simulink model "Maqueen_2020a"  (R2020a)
settings: Solver=VariableStepAuto  StartTime=0.0  StopTime=2  RelTol=1e-3
model workspace: external: MAT-File (data not in the file)
undefined symbols (not defined in the file or in its folder): deg, kg, m, mm, N, rad, s, smiData, X, Y, Z
libraries: sm_lib x459, fl_lib x12, nesl_utility x10
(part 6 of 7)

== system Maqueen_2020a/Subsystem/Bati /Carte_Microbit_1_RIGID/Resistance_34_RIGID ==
  ReferenceFrame : sm_lib/Frames and Transforms/Reference Frame
  Solid : sm_lib/Body Elements/File Solid  ExtGeomFileName=Resistance_Defaut_sldprt.STL  UnitType=Custom  ExtGeomFileUnits=mm  StepReaderType=HEX  ExportConvexHullGeometry=off  InertiaType=Custom  Mass=smiData.Solid(7).mass  MassUnits=kg  CenterOfMass=smiData.Solid(7).CoM  CenterOfMassUnits=mm  MomentsOfInertia=smiData.Solid(7).MoI  MomentsOfInertiaUnits=kg*mm^2  ProductsOfInertia=smiData.Solid(7).PoI  ProductsOfInertiaUnits=kg*mm^2  BasedOnType=Density  Density=1000  DensityUnits=kg/m^3  DoExposeReferenceFrame=on  SerializedFrames=<Frames/>  GraphicType=FromGeometry  MarkerShape=Sphere  MarkerSize=10  GraphicVisPropType=SimpleVisualProperties  GraphicDiffuseColor=smiData.Solid(7).color  GraphicSpecularColor=[0.5 0.5 0.5 1.0]  GraphicAmbientColor=[0.15 0.15 0.15 1.0]  GraphicEmissiveColor=[0.0 0.0 0.0 1.0]  GraphicShininess=75  GraphicOpacity=smiData.Solid(7).opacity
  F : PMIOPort  Side=Left
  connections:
  ReferenceFrame/RConn1 -- Solid/RConn1 -- F/RConn1

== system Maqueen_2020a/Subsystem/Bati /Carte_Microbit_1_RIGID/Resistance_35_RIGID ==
  ReferenceFrame : sm_lib/Frames and Transforms/Reference Frame
  Solid : sm_lib/Body Elements/File Solid  ExtGeomFileName=Resistance_Defaut_sldprt.STL  UnitType=Custom  ExtGeomFileUnits=mm  StepReaderType=HEX  ExportConvexHullGeometry=off  InertiaType=Custom  Mass=smiData.Solid(7).mass  MassUnits=kg  CenterOfMass=smiData.Solid(7).CoM  CenterOfMassUnits=mm  MomentsOfInertia=smiData.Solid(7).MoI  MomentsOfInertiaUnits=kg*mm^2  ProductsOfInertia=smiData.Solid(7).PoI  ProductsOfInertiaUnits=kg*mm^2  BasedOnType=Density  Density=1000  DensityUnits=kg/m^3  DoExposeReferenceFrame=on  SerializedFrames=<Frames/>  GraphicType=FromGeometry  MarkerShape=Sphere  MarkerSize=10  GraphicVisPropType=SimpleVisualProperties  GraphicDiffuseColor=smiData.Solid(7).color  GraphicSpecularColor=[0.5 0.5 0.5 1.0]  GraphicAmbientColor=[0.15 0.15 0.15 1.0]  GraphicEmissiveColor=[0.0 0.0 0.0 1.0]  GraphicShininess=75  GraphicOpacity=smiData.Solid(7).opacity
  F : PMIOPort  Side=Left
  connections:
  ReferenceFrame/RConn1 -- Solid/RConn1 -- F/RConn1

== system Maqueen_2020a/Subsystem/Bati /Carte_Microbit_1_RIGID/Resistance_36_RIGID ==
  ReferenceFrame : sm_lib/Frames and Transforms/Reference Frame
  Solid : sm_lib/Body Elements/File Solid  ExtGeomFileName=Resistance_Defaut_sldprt.STL  UnitType=Custom  ExtGeomFileUnits=mm  StepReaderType=HEX  ExportConvexHullGeometry=off  InertiaType=Custom  Mass=smiData.Solid(7).mass  MassUnits=kg  CenterOfMass=smiData.Solid(7).CoM  CenterOfMassUnits=mm  MomentsOfInertia=smiData.Solid(7).MoI  MomentsOfInertiaUnits=kg*mm^2  ProductsOfInertia=smiData.Solid(7).PoI  ProductsOfInertiaUnits=kg*mm^2  BasedOnType=Density  Density=1000  DensityUnits=kg/m^3  DoExposeReferenceFrame=on  SerializedFrames=<Frames/>  GraphicType=FromGeometry  MarkerShape=Sphere  MarkerSize=10  GraphicVisPropType=SimpleVisualProperties  GraphicDiffuseColor=smiData.Solid(7).color  GraphicSpecularColor=[0.5 0.5 0.5 1.0]  GraphicAmbientColor=[0.15 0.15 0.15 1.0]  GraphicEmissiveColor=[0.0 0.0 0.0 1.0]  GraphicShininess=75  GraphicOpacity=smiData.Solid(7).opacity
  F : PMIOPort  Side=Left
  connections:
  ReferenceFrame/RConn1 -- Solid/RConn1 -- F/RConn1

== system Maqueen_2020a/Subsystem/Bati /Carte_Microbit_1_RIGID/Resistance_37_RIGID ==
  ReferenceFrame : sm_lib/Frames and Transforms/Reference Frame
  Solid : sm_lib/Body Elements/File Solid  ExtGeomFileName=Resistance_Defaut_sldprt.STL  UnitType=Custom  ExtGeomFileUnits=mm  StepReaderType=HEX  ExportConvexHullGeometry=off  InertiaType=Custom  Mass=smiData.Solid(7).mass  MassUnits=kg  CenterOfMass=smiData.Solid(7).CoM  CenterOfMassUnits=mm  MomentsOfInertia=smiData.Solid(7).MoI  MomentsOfInertiaUnits=kg*mm^2  ProductsOfInertia=smiData.Solid(7).PoI  ProductsOfInertiaUnits=kg*mm^2  BasedOnType=Density  Density=1000  DensityUnits=kg/m^3  DoExposeReferenceFrame=on  SerializedFrames=<Frames/>  GraphicType=FromGeometry  MarkerShape=Sphere  MarkerSize=10  GraphicVisPropType=SimpleVisualProperties  GraphicDiffuseColor=smiData.Solid(7).color  GraphicSpecularColor=[0.5 0.5 0.5 1.0]  GraphicAmbientColor=[0.15 0.15 0.15 1.0]  GraphicEmissiveColor=[0.0 0.0 0.0 1.0]  GraphicShininess=75  GraphicOpacity=smiData.Solid(7).opacity
  F : PMIOPort  Side=Left
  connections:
  ReferenceFrame/RConn1 -- Solid/RConn1 -- F/RConn1

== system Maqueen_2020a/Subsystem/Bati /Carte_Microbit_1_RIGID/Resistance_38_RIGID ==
  ReferenceFrame : sm_lib/Frames and Transforms/Reference Frame
  Solid : sm_lib/Body Elements/File Solid  ExtGeomFileName=Resistance_Defaut_sldprt.STL  UnitType=Custom  ExtGeomFileUnits=mm  StepReaderType=HEX  ExportConvexHullGeometry=off  InertiaType=Custom  Mass=smiData.Solid(7).mass  MassUnits=kg  CenterOfMass=smiData.Solid(7).CoM  CenterOfMassUnits=mm  MomentsOfInertia=smiData.Solid(7).MoI  MomentsOfInertiaUnits=kg*mm^2  ProductsOfInertia=smiData.Solid(7).PoI  ProductsOfInertiaUnits=kg*mm^2  BasedOnType=Density  Density=1000  DensityUnits=kg/m^3  DoExposeReferenceFrame=on  SerializedFrames=<Frames/>  GraphicType=FromGeometry  MarkerShape=Sphere  MarkerSize=10  GraphicVisPropType=SimpleVisualProperties  GraphicDiffuseColor=smiData.Solid(7).color  GraphicSpecularColor=[0.5 0.5 0.5 1.0]  GraphicAmbientColor=[0.15 0.15 0.15 1.0]  GraphicEmissiveColor=[0.0 0.0 0.0 1.0]  GraphicShininess=75  GraphicOpacity=smiData.Solid(7).opacity
  F : PMIOPort  Side=Left
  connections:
  ReferenceFrame/RConn1 -- Solid/RConn1 -- F/RConn1

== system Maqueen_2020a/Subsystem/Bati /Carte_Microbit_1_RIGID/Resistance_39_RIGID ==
  ReferenceFrame : sm_lib/Frames and Transforms/Reference Frame
  Solid : sm_lib/Body Elements/File Solid  ExtGeomFileName=Resistance_Defaut_sldprt.STL  UnitType=Custom  ExtGeomFileUnits=mm  StepReaderType=HEX  ExportConvexHullGeometry=off  InertiaType=Custom  Mass=smiData.Solid(7).mass  MassUnits=kg  CenterOfMass=smiData.Solid(7).CoM  CenterOfMassUnits=mm  MomentsOfInertia=smiData.Solid(7).MoI  MomentsOfInertiaUnits=kg*mm^2  ProductsOfInertia=smiData.Solid(7).PoI  ProductsOfInertiaUnits=kg*mm^2  BasedOnType=Density  Density=1000  DensityUnits=kg/m^3  DoExposeReferenceFrame=on  SerializedFrames=<Frames/>  GraphicType=FromGeometry  MarkerShape=Sphere  MarkerSize=10  GraphicVisPropType=SimpleVisualProperties  GraphicDiffuseColor=smiData.Solid(7).color  GraphicSpecularColor=[0.5 0.5 0.5 1.0]  GraphicAmbientColor=[0.15 0.15 0.15 1.0]  GraphicEmissiveColor=[0.0 0.0 0.0 1.0]  GraphicShininess=75  GraphicOpacity=smiData.Solid(7).opacity
  F : PMIOPort  Side=Left
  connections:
  ReferenceFrame/RConn1 -- Solid/RConn1 -- F/RConn1

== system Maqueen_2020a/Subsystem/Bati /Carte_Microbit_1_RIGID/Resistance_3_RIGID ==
  ReferenceFrame : sm_lib/Frames and Transforms/Reference Frame
  Solid : sm_lib/Body Elements/File Solid  ExtGeomFileName=Resistance_Defaut_sldprt.STL  UnitType=Custom  ExtGeomFileUnits=mm  StepReaderType=HEX  ExportConvexHullGeometry=off  InertiaType=Custom  Mass=smiData.Solid(7).mass  MassUnits=kg  CenterOfMass=smiData.Solid(7).CoM  CenterOfMassUnits=mm  MomentsOfInertia=smiData.Solid(7).MoI  MomentsOfInertiaUnits=kg*mm^2  ProductsOfInertia=smiData.Solid(7).PoI  ProductsOfInertiaUnits=kg*mm^2  BasedOnType=Density  Density=1000  DensityUnits=kg/m^3  DoExposeReferenceFrame=on  SerializedFrames=<Frames/>  GraphicType=FromGeometry  MarkerShape=Sphere  MarkerSize=10  GraphicVisPropType=SimpleVisualProperties  GraphicDiffuseColor=smiData.Solid(7).color  GraphicSpecularColor=[0.5 0.5 0.5 1.0]  GraphicAmbientColor=[0.15 0.15 0.15 1.0]  GraphicEmissiveColor=[0.0 0.0 0.0 1.0]  GraphicShininess=75  GraphicOpacity=smiData.Solid(7).opacity
  F : PMIOPort  Side=Left
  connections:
  ReferenceFrame/RConn1 -- Solid/RConn1 -- F/RConn1

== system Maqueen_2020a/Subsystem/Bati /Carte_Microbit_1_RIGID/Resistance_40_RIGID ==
  ReferenceFrame : sm_lib/Frames and Transforms/Reference Frame
  Solid : sm_lib/Body Elements/File Solid  ExtGeomFileName=Resistance_Defaut_sldprt.STL  UnitType=Custom  ExtGeomFileUnits=mm  StepReaderType=HEX  ExportConvexHullGeometry=off  InertiaType=Custom  Mass=smiData.Solid(7).mass  MassUnits=kg  CenterOfMass=smiData.Solid(7).CoM  CenterOfMassUnits=mm  MomentsOfInertia=smiData.Solid(7).MoI  MomentsOfInertiaUnits=kg*mm^2  ProductsOfInertia=smiData.Solid(7).PoI  ProductsOfInertiaUnits=kg*mm^2  BasedOnType=Density  Density=1000  DensityUnits=kg/m^3  DoExposeReferenceFrame=on  SerializedFrames=<Frames/>  GraphicType=FromGeometry  MarkerShape=Sphere  MarkerSize=10  GraphicVisPropType=SimpleVisualProperties  GraphicDiffuseColor=smiData.Solid(7).color  GraphicSpecularColor=[0.5 0.5 0.5 1.0]  GraphicAmbientColor=[0.15 0.15 0.15 1.0]  GraphicEmissiveColor=[0.0 0.0 0.0 1.0]  GraphicShininess=75  GraphicOpacity=smiData.Solid(7).opacity
  F : PMIOPort  Side=Left
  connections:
  ReferenceFrame/RConn1 -- Solid/RConn1 -- F/RConn1

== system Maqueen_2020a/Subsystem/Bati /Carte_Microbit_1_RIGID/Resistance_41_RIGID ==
  ReferenceFrame : sm_lib/Frames and Transforms/Reference Frame
  Solid : sm_lib/Body Elements/File Solid  ExtGeomFileName=Resistance_Defaut_sldprt.STL  UnitType=Custom  ExtGeomFileUnits=mm  StepReaderType=HEX  ExportConvexHullGeometry=off  InertiaType=Custom  Mass=smiData.Solid(7).mass  MassUnits=kg  CenterOfMass=smiData.Solid(7).CoM  CenterOfMassUnits=mm  MomentsOfInertia=smiData.Solid(7).MoI  MomentsOfInertiaUnits=kg*mm^2  ProductsOfInertia=smiData.Solid(7).PoI  ProductsOfInertiaUnits=kg*mm^2  BasedOnType=Density  Density=1000  DensityUnits=kg/m^3  DoExposeReferenceFrame=on  SerializedFrames=<Frames/>  GraphicType=FromGeometry  MarkerShape=Sphere  MarkerSize=10  GraphicVisPropType=SimpleVisualProperties  GraphicDiffuseColor=smiData.Solid(7).color  GraphicSpecularColor=[0.5 0.5 0.5 1.0]  GraphicAmbientColor=[0.15 0.15 0.15 1.0]  GraphicEmissiveColor=[0.0 0.0 0.0 1.0]  GraphicShininess=75  GraphicOpacity=smiData.Solid(7).opacity
  F : PMIOPort  Side=Left
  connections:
  ReferenceFrame/RConn1 -- Solid/RConn1 -- F/RConn1

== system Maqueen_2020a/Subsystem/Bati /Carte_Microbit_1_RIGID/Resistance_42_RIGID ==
  ReferenceFrame : sm_lib/Frames and Transforms/Reference Frame
  Solid : sm_lib/Body Elements/File Solid  ExtGeomFileName=Resistance_Defaut_sldprt.STL  UnitType=Custom  ExtGeomFileUnits=mm  StepReaderType=HEX  ExportConvexHullGeometry=off  InertiaType=Custom  Mass=smiData.Solid(7).mass  MassUnits=kg  CenterOfMass=smiData.Solid(7).CoM  CenterOfMassUnits=mm  MomentsOfInertia=smiData.Solid(7).MoI  MomentsOfInertiaUnits=kg*mm^2  ProductsOfInertia=smiData.Solid(7).PoI  ProductsOfInertiaUnits=kg*mm^2  BasedOnType=Density  Density=1000  DensityUnits=kg/m^3  DoExposeReferenceFrame=on  SerializedFrames=<Frames/>  GraphicType=FromGeometry  MarkerShape=Sphere  MarkerSize=10  GraphicVisPropType=SimpleVisualProperties  GraphicDiffuseColor=smiData.Solid(7).color  GraphicSpecularColor=[0.5 0.5 0.5 1.0]  GraphicAmbientColor=[0.15 0.15 0.15 1.0]  GraphicEmissiveColor=[0.0 0.0 0.0 1.0]  GraphicShininess=75  GraphicOpacity=smiData.Solid(7).opacity
  F : PMIOPort  Side=Left
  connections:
  ReferenceFrame/RConn1 -- Solid/RConn1 -- F/RConn1

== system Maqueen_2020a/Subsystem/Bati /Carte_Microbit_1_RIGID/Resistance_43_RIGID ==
  ReferenceFrame : sm_lib/Frames and Transforms/Reference Frame
  Solid : sm_lib/Body Elements/File Solid  ExtGeomFileName=Resistance_Defaut_sldprt.STL  UnitType=Custom  ExtGeomFileUnits=mm  StepReaderType=HEX  ExportConvexHullGeometry=off  InertiaType=Custom  Mass=smiData.Solid(7).mass  MassUnits=kg  CenterOfMass=smiData.Solid(7).CoM  CenterOfMassUnits=mm  MomentsOfInertia=smiData.Solid(7).MoI  MomentsOfInertiaUnits=kg*mm^2  ProductsOfInertia=smiData.Solid(7).PoI  ProductsOfInertiaUnits=kg*mm^2  BasedOnType=Density  Density=1000  DensityUnits=kg/m^3  DoExposeReferenceFrame=on  SerializedFrames=<Frames/>  GraphicType=FromGeometry  MarkerShape=Sphere  MarkerSize=10  GraphicVisPropType=SimpleVisualProperties  GraphicDiffuseColor=smiData.Solid(7).color  GraphicSpecularColor=[0.5 0.5 0.5 1.0]  GraphicAmbientColor=[0.15 0.15 0.15 1.0]  GraphicEmissiveColor=[0.0 0.0 0.0 1.0]  GraphicShininess=75  GraphicOpacity=smiData.Solid(7).opacity
  F : PMIOPort  Side=Left
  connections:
  ReferenceFrame/RConn1 -- Solid/RConn1 -- F/RConn1

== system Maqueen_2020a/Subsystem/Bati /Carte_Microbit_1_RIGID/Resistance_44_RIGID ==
  ReferenceFrame : sm_lib/Frames and Transforms/Reference Frame
  Solid : sm_lib/Body Elements/File Solid  ExtGeomFileName=Resistance_Defaut_sldprt.STL  UnitType=Custom  ExtGeomFileUnits=mm  StepReaderType=HEX  ExportConvexHullGeometry=off  InertiaType=Custom  Mass=smiData.Solid(7).mass  MassUnits=kg  CenterOfMass=smiData.Solid(7).CoM  CenterOfMassUnits=mm  MomentsOfInertia=smiData.Solid(7).MoI  MomentsOfInertiaUnits=kg*mm^2  ProductsOfInertia=smiData.Solid(7).PoI  ProductsOfInertiaUnits=kg*mm^2  BasedOnType=Density  Density=1000  DensityUnits=kg/m^3  DoExposeReferenceFrame=on  SerializedFrames=<Frames/>  GraphicType=FromGeometry  MarkerShape=Sphere  MarkerSize=10  GraphicVisPropType=SimpleVisualProperties  GraphicDiffuseColor=smiData.Solid(7).color  GraphicSpecularColor=[0.5 0.5 0.5 1.0]  GraphicAmbientColor=[0.15 0.15 0.15 1.0]  GraphicEmissiveColor=[0.0 0.0 0.0 1.0]  GraphicShininess=75  GraphicOpacity=smiData.Solid(7).opacity
  F : PMIOPort  Side=Left
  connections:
  ReferenceFrame/RConn1 -- Solid/RConn1 -- F/RConn1

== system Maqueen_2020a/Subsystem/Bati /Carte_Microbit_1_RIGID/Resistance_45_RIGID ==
  ReferenceFrame : sm_lib/Frames and Transforms/Reference Frame
  Solid : sm_lib/Body Elements/File Solid  ExtGeomFileName=Resistance_Defaut_sldprt.STL  UnitType=Custom  ExtGeomFileUnits=mm  StepReaderType=HEX  ExportConvexHullGeometry=off  InertiaType=Custom  Mass=smiData.Solid(7).mass  MassUnits=kg  CenterOfMass=smiData.Solid(7).CoM  CenterOfMassUnits=mm  MomentsOfInertia=smiData.Solid(7).MoI  MomentsOfInertiaUnits=kg*mm^2  ProductsOfInertia=smiData.Solid(7).PoI  ProductsOfInertiaUnits=kg*mm^2  BasedOnType=Density  Density=1000  DensityUnits=kg/m^3  DoExposeReferenceFrame=on  SerializedFrames=<Frames/>  GraphicType=FromGeometry  MarkerShape=Sphere  MarkerSize=10  GraphicVisPropType=SimpleVisualProperties  GraphicDiffuseColor=smiData.Solid(7).color  GraphicSpecularColor=[0.5 0.5 0.5 1.0]  GraphicAmbientColor=[0.15 0.15 0.15 1.0]  GraphicEmissiveColor=[0.0 0.0 0.0 1.0]  GraphicShininess=75  GraphicOpacity=smiData.Solid(7).opacity
  F : PMIOPort  Side=Left
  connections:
  ReferenceFrame/RConn1 -- Solid/RConn1 -- F/RConn1

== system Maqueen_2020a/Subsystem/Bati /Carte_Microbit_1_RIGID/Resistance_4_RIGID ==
  ReferenceFrame : sm_lib/Frames and Transforms/Reference Frame
  Solid : sm_lib/Body Elements/File Solid  ExtGeomFileName=Resistance_Defaut_sldprt.STL  UnitType=Custom  ExtGeomFileUnits=mm  StepReaderType=HEX  ExportConvexHullGeometry=off  InertiaType=Custom  Mass=smiData.Solid(7).mass  MassUnits=kg  CenterOfMass=smiData.Solid(7).CoM  CenterOfMassUnits=mm  MomentsOfInertia=smiData.Solid(7).MoI  MomentsOfInertiaUnits=kg*mm^2  ProductsOfInertia=smiData.Solid(7).PoI  ProductsOfInertiaUnits=kg*mm^2  BasedOnType=Density  Density=1000  DensityUnits=kg/m^3  DoExposeReferenceFrame=on  SerializedFrames=<Frames/>  GraphicType=FromGeometry  MarkerShape=Sphere  MarkerSize=10  GraphicVisPropType=SimpleVisualProperties  GraphicDiffuseColor=smiData.Solid(7).color  GraphicSpecularColor=[0.5 0.5 0.5 1.0]  GraphicAmbientColor=[0.15 0.15 0.15 1.0]  GraphicEmissiveColor=[0.0 0.0 0.0 1.0]  GraphicShininess=75  GraphicOpacity=smiData.Solid(7).opacity
  F : PMIOPort  Side=Left
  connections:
  ReferenceFrame/RConn1 -- Solid/RConn1 -- F/RConn1

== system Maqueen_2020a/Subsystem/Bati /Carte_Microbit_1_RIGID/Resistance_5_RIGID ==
  ReferenceFrame : sm_lib/Frames and Transforms/Reference Frame
  Solid : sm_lib/Body Elements/File Solid  ExtGeomFileName=Resistance_Defaut_sldprt.STL  UnitType=Custom  ExtGeomFileUnits=mm  StepReaderType=HEX  ExportConvexHullGeometry=off  InertiaType=Custom  Mass=smiData.Solid(7).mass  MassUnits=kg  CenterOfMass=smiData.Solid(7).CoM  CenterOfMassUnits=mm  MomentsOfInertia=smiData.Solid(7).MoI  MomentsOfInertiaUnits=kg*mm^2  ProductsOfInertia=smiData.Solid(7).PoI  ProductsOfInertiaUnits=kg*mm^2  BasedOnType=Density  Density=1000  DensityUnits=kg/m^3  DoExposeReferenceFrame=on  SerializedFrames=<Frames/>  GraphicType=FromGeometry  MarkerShape=Sphere  MarkerSize=10  GraphicVisPropType=SimpleVisualProperties  GraphicDiffuseColor=smiData.Solid(7).color  GraphicSpecularColor=[0.5 0.5 0.5 1.0]  GraphicAmbientColor=[0.15 0.15 0.15 1.0]  GraphicEmissiveColor=[0.0 0.0 0.0 1.0]  GraphicShininess=75  GraphicOpacity=smiData.Solid(7).opacity
  F : PMIOPort  Side=Left
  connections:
  ReferenceFrame/RConn1 -- Solid/RConn1 -- F/RConn1

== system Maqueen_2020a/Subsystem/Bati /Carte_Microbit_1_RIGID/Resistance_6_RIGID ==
  ReferenceFrame : sm_lib/Frames and Transforms/Reference Frame
  Solid : sm_lib/Body Elements/File Solid  ExtGeomFileName=Resistance_Defaut_sldprt.STL  UnitType=Custom  ExtGeomFileUnits=mm  StepReaderType=HEX  ExportConvexHullGeometry=off  InertiaType=Custom  Mass=smiData.Solid(7).mass  MassUnits=kg  CenterOfMass=smiData.Solid(7).CoM  CenterOfMassUnits=mm  MomentsOfInertia=smiData.Solid(7).MoI  MomentsOfInertiaUnits=kg*mm^2  ProductsOfInertia=smiData.Solid(7).PoI  ProductsOfInertiaUnits=kg*mm^2  BasedOnType=Density  Density=1000  DensityUnits=kg/m^3  DoExposeReferenceFrame=on  SerializedFrames=<Frames/>  GraphicType=FromGeometry  MarkerShape=Sphere  MarkerSize=10  GraphicVisPropType=SimpleVisualProperties  GraphicDiffuseColor=smiData.Solid(7).color  GraphicSpecularColor=[0.5 0.5 0.5 1.0]  GraphicAmbientColor=[0.15 0.15 0.15 1.0]  GraphicEmissiveColor=[0.0 0.0 0.0 1.0]  GraphicShininess=75  GraphicOpacity=smiData.Solid(7).opacity
  F : PMIOPort  Side=Left
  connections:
  ReferenceFrame/RConn1 -- Solid/RConn1 -- F/RConn1

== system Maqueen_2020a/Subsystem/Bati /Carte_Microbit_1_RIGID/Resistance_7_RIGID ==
  ReferenceFrame : sm_lib/Frames and Transforms/Reference Frame
  Solid : sm_lib/Body Elements/File Solid  ExtGeomFileName=Resistance_Defaut_sldprt.STL  UnitType=Custom  ExtGeomFileUnits=mm  StepReaderType=HEX  ExportConvexHullGeometry=off  InertiaType=Custom  Mass=smiData.Solid(7).mass  MassUnits=kg  CenterOfMass=smiData.Solid(7).CoM  CenterOfMassUnits=mm  MomentsOfInertia=smiData.Solid(7).MoI  MomentsOfInertiaUnits=kg*mm^2  ProductsOfInertia=smiData.Solid(7).PoI  ProductsOfInertiaUnits=kg*mm^2  BasedOnType=Density  Density=1000  DensityUnits=kg/m^3  DoExposeReferenceFrame=on  SerializedFrames=<Frames/>  GraphicType=FromGeometry  MarkerShape=Sphere  MarkerSize=10  GraphicVisPropType=SimpleVisualProperties  GraphicDiffuseColor=smiData.Solid(7).color  GraphicSpecularColor=[0.5 0.5 0.5 1.0]  GraphicAmbientColor=[0.15 0.15 0.15 1.0]  GraphicEmissiveColor=[0.0 0.0 0.0 1.0]  GraphicShininess=75  GraphicOpacity=smiData.Solid(7).opacity
  F : PMIOPort  Side=Left
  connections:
  ReferenceFrame/RConn1 -- Solid/RConn1 -- F/RConn1

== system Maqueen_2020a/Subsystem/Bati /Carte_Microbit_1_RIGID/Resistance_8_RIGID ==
  ReferenceFrame : sm_lib/Frames and Transforms/Reference Frame
  Solid : sm_lib/Body Elements/File Solid  ExtGeomFileName=Resistance_Defaut_sldprt.STL  UnitType=Custom  ExtGeomFileUnits=mm  StepReaderType=HEX  ExportConvexHullGeometry=off  InertiaType=Custom  Mass=smiData.Solid(7).mass  MassUnits=kg  CenterOfMass=smiData.Solid(7).CoM  CenterOfMassUnits=mm  MomentsOfInertia=smiData.Solid(7).MoI  MomentsOfInertiaUnits=kg*mm^2  ProductsOfInertia=smiData.Solid(7).PoI  ProductsOfInertiaUnits=kg*mm^2  BasedOnType=Density  Density=1000  DensityUnits=kg/m^3  DoExposeReferenceFrame=on  SerializedFrames=<Frames/>  GraphicType=FromGeometry  MarkerShape=Sphere  MarkerSize=10  GraphicVisPropType=SimpleVisualProperties  GraphicDiffuseColor=smiData.Solid(7).color  GraphicSpecularColor=[0.5 0.5 0.5 1.0]  GraphicAmbientColor=[0.15 0.15 0.15 1.0]  GraphicEmissiveColor=[0.0 0.0 0.0 1.0]  GraphicShininess=75  GraphicOpacity=smiData.Solid(7).opacity
  F : PMIOPort  Side=Left
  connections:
  ReferenceFrame/RConn1 -- Solid/RConn1 -- F/RConn1

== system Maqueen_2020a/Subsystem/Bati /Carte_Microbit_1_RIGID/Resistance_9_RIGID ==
  ReferenceFrame : sm_lib/Frames and Transforms/Reference Frame
  Solid : sm_lib/Body Elements/File Solid  ExtGeomFileName=Resistance_Defaut_sldprt.STL  UnitType=Custom  ExtGeomFileUnits=mm  StepReaderType=HEX  ExportConvexHullGeometry=off  InertiaType=Custom  Mass=smiData.Solid(7).mass  MassUnits=kg  CenterOfMass=smiData.Solid(7).CoM  CenterOfMassUnits=mm  MomentsOfInertia=smiData.Solid(7).MoI  MomentsOfInertiaUnits=kg*mm^2  ProductsOfInertia=smiData.Solid(7).PoI  ProductsOfInertiaUnits=kg*mm^2  BasedOnType=Density  Density=1000  DensityUnits=kg/m^3  DoExposeReferenceFrame=on  SerializedFrames=<Frames/>  GraphicType=FromGeometry  MarkerShape=Sphere  MarkerSize=10  GraphicVisPropType=SimpleVisualProperties  GraphicDiffuseColor=smiData.Solid(7).color  GraphicSpecularColor=[0.5 0.5 0.5 1.0]  GraphicAmbientColor=[0.15 0.15 0.15 1.0]  GraphicEmissiveColor=[0.0 0.0 0.0 1.0]  GraphicShininess=75  GraphicOpacity=smiData.Solid(7).opacity
  F : PMIOPort  Side=Left
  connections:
  ReferenceFrame/RConn1 -- Solid/RConn1 -- F/RConn1

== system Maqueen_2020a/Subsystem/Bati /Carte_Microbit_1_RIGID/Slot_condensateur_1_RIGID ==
  ReferenceFrame : sm_lib/Frames and Transforms/Reference Frame
  Solid : sm_lib/Body Elements/File Solid  ExtGeomFileName=Slot condensateur_Defaut_sldprt.STL  UnitType=Custom  ExtGeomFileUnits=mm  StepReaderType=HEX  ExportConvexHullGeometry=off  InertiaType=Custom  Mass=smiData.Solid(22).mass  MassUnits=kg  CenterOfMass=smiData.Solid(22).CoM  CenterOfMassUnits=mm  MomentsOfInertia=smiData.Solid(22).MoI  MomentsOfInertiaUnits=kg*mm^2  ProductsOfInertia=smiData.Solid(22).PoI  ProductsOfInertiaUnits=kg*mm^2  BasedOnType=Density  Density=1000  DensityUnits=kg/m^3  DoExposeReferenceFrame=on  SerializedFrames=<Frames/>  GraphicType=FromGeometry  MarkerShape=Sphere  MarkerSize=10  GraphicVisPropType=SimpleVisualProperties  GraphicDiffuseColor=smiData.Solid(22).color  GraphicSpecularColor=[0.5 0.5 0.5 1.0]  GraphicAmbientColor=[0.15 0.15 0.15 1.0]  GraphicEmissiveColor=[0.0 0.0 0.0 1.0]  GraphicShininess=75  GraphicOpacity=smiData.Solid(22).opacity
  F : PMIOPort  Side=Left
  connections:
  ReferenceFrame/RConn1 -- Solid/RConn1 -- F/RConn1

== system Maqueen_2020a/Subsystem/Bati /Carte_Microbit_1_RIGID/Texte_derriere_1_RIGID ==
  ReferenceFrame : sm_lib/Frames and Transforms/Reference Frame
  Solid : sm_lib/Body Elements/File Solid  ExtGeomFileName=Texte derriere_Defaut_sldprt.STL  UnitType=Custom  ExtGeomFileUnits=mm  StepReaderType=HEX  ExportConvexHullGeometry=off  InertiaType=Custom  Mass=smiData.Solid(19).mass  MassUnits=kg  CenterOfMass=smiData.Solid(19).CoM  CenterOfMassUnits=mm  MomentsOfInertia=smiData.Solid(19).MoI  MomentsOfInertiaUnits=kg*mm^2  ProductsOfInertia=smiData.Solid(19).PoI  ProductsOfInertiaUnits=kg*mm^2  BasedOnType=Density  Density=1000  DensityUnits=kg/m^3  DoExposeReferenceFrame=on  SerializedFrames=<Frames/>  GraphicType=FromGeometry  MarkerShape=Sphere  MarkerSize=10  GraphicVisPropType=SimpleVisualProperties  GraphicDiffuseColor=smiData.Solid(19).color  GraphicSpecularColor=[0.5 0.5 0.5 1.0]  GraphicAmbientColor=[0.15 0.15 0.15 1.0]  GraphicEmissiveColor=[0.0 0.0 0.0 1.0]  GraphicShininess=75  GraphicOpacity=smiData.Solid(19).opacity
  F : PMIOPort  Side=Left
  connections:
  ReferenceFrame/RConn1 -- Solid/RConn1 -- F/RConn1

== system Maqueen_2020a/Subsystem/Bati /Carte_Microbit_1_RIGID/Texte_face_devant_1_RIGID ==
  ReferenceFrame : sm_lib/Frames and Transforms/Reference Frame
  Solid : sm_lib/Body Elements/File Solid  ExtGeomFileName=Texte face devant_Defaut_sldprt.STL  UnitType=Custom  ExtGeomFileUnits=mm  StepReaderType=HEX  ExportConvexHullGeometry=off  InertiaType=Custom  Mass=smiData.Solid(15).mass  MassUnits=kg  CenterOfMass=smiData.Solid(15).CoM  CenterOfMassUnits=mm  MomentsOfInertia=smiData.Solid(15).MoI  MomentsOfInertiaUnits=kg*mm^2  ProductsOfInertia=smiData.Solid(15).PoI  ProductsOfInertiaUnits=kg*mm^2  BasedOnType=Density  Density=1000  DensityUnits=kg/m^3  DoExposeReferenceFrame=on  SerializedFrames=<Frames/>  GraphicType=FromGeometry  MarkerShape=Sphere  MarkerSize=10  GraphicVisPropType=SimpleVisualProperties  GraphicDiffuseColor=smiData.Solid(15).color  GraphicSpecularColor=[0.5 0.5 0.5 1.0]  GraphicAmbientColor=[0.15 0.15 0.15 1.0]  GraphicEmissiveColor=[0.0 0.0 0.0 1.0]  GraphicShininess=75  GraphicOpacity=smiData.Solid(15).opacity
  F : PMIOPort  Side=Left
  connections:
  ReferenceFrame/RConn1 -- Solid/RConn1 -- F/RConn1

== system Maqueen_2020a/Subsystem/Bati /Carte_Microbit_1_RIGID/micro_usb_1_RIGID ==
  ReferenceFrame : sm_lib/Frames and Transforms/Reference Frame
  Solid : sm_lib/Body Elements/File Solid  ExtGeomFileName=micro usb_Defaut_sldprt.STL  UnitType=Custom  ExtGeomFileUnits=mm  StepReaderType=HEX  ExportConvexHullGeometry=off  InertiaType=Custom  Mass=smiData.Solid(18).mass  MassUnits=kg  CenterOfMass=smiData.Solid(18).CoM  CenterOfMassUnits=mm  MomentsOfInertia=smiData.Solid(18).MoI  MomentsOfInertiaUnits=kg*mm^2  ProductsOfInertia=smiData.Solid(18).PoI  ProductsOfInertiaUnits=kg*mm^2  BasedOnType=Density  Density=1000  DensityUnits=kg/m^3  DoExposeReferenceFrame=on  SerializedFrames=<Frames/>  GraphicType=FromGeometry  MarkerShape=Sphere  MarkerSize=10  GraphicVisPropType=SimpleVisualProperties  GraphicDiffuseColor=smiData.Solid(18).color  GraphicSpecularColor=[0.5 0.5 0.5 1.0]  GraphicAmbientColor=[0.15 0.15 0.15 1.0]  GraphicEmissiveColor=[0.0 0.0 0.0 1.0]  GraphicShininess=75  GraphicOpacity=smiData.Solid(18).opacity
  F : PMIOPort  Side=Left
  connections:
  ReferenceFrame/RConn1 -- Solid/RConn1 -- F/RConn1

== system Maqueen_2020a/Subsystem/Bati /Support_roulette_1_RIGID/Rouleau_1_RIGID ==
  ReferenceFrame : sm_lib/Frames and Transforms/Reference Frame
  Solid : sm_lib/Body Elements/File Solid  ExtGeomFileName=Rouleau_Defaut_sldprt.STL  UnitType=Custom  ExtGeomFileUnits=mm  StepReaderType=HEX  ExportConvexHullGeometry=off  InertiaType=Custom  Mass=smiData.Solid(31).mass  MassUnits=kg  CenterOfMass=smiData.Solid(31).CoM  CenterOfMassUnits=mm  MomentsOfInertia=smiData.Solid(31).MoI  MomentsOfInertiaUnits=kg*mm^2  ProductsOfInertia=smiData.Solid(31).PoI  ProductsOfInertiaUnits=kg*mm^2  BasedOnType=Density  Density=1000  DensityUnits=kg/m^3  DoExposeReferenceFrame=on  SerializedFrames=<Frames/>  GraphicType=FromGeometry  MarkerShape=Sphere  MarkerSize=10  GraphicVisPropType=SimpleVisualProperties  GraphicDiffuseColor=smiData.Solid(31).color  GraphicSpecularColor=[0.5 0.5 0.5 1.0]  GraphicAmbientColor=[0.15 0.15 0.15 1.0]  GraphicEmissiveColor=[0.0 0.0 0.0 1.0]  GraphicShininess=75  GraphicOpacity=smiData.Solid(31).opacity
  F : PMIOPort  Side=Left
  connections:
  ReferenceFrame/RConn1 -- Solid/RConn1 -- F/RConn1

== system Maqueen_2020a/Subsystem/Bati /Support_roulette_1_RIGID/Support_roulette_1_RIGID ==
  ReferenceFrame : sm_lib/Frames and Transforms/Reference Frame
  Solid : sm_lib/Body Elements/File Solid  ExtGeomFileName=Support roulette_Defaut_sldprt.STL  UnitType=Custom  ExtGeomFileUnits=mm  StepReaderType=HEX  ExportConvexHullGeometry=off  InertiaType=Custom  Mass=smiData.Solid(30).mass  MassUnits=kg  CenterOfMass=smiData.Solid(30).CoM  CenterOfMassUnits=mm  MomentsOfInertia=smiData.Solid(30).MoI  MomentsOfInertiaUnits=kg*mm^2  ProductsOfInertia=smiData.Solid(30).PoI  ProductsOfInertiaUnits=kg*mm^2  BasedOnType=Density  Density=1000  DensityUnits=kg/m^3  DoExposeReferenceFrame=on  SerializedFrames=<Frames/>  GraphicType=FromGeometry  MarkerShape=Sphere  MarkerSize=10  GraphicVisPropType=SimpleVisualProperties  GraphicDiffuseColor=smiData.Solid(30).color  GraphicSpecularColor=[0.5 0.5 0.5 1.0]  GraphicAmbientColor=[0.15 0.15 0.15 1.0]  GraphicEmissiveColor=[0.0 0.0 0.0 1.0]  GraphicShininess=75  GraphicOpacity=smiData.Solid(30).opacity
  F : PMIOPort  Side=Left
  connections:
  ReferenceFrame/RConn1 -- Solid/RConn1 -- F/RConn1

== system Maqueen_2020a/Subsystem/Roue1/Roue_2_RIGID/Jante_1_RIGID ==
  ReferenceFrame : sm_lib/Frames and Transforms/Reference Frame
  Solid : sm_lib/Body Elements/File Solid  ExtGeomFileName=Jante_Defaut_sldprt.STL  UnitType=Custom  ExtGeomFileUnits=mm  StepReaderType=HEX  ExportConvexHullGeometry=off  InertiaType=Custom  Mass=smiData.Solid(3).mass  MassUnits=kg  CenterOfMass=smiData.Solid(3).CoM  CenterOfMassUnits=mm  MomentsOfInertia=smiData.Solid(3).MoI  MomentsOfInertiaUnits=kg*mm^2  ProductsOfInertia=smiData.Solid(3).PoI  ProductsOfInertiaUnits=kg*mm^2  BasedOnType=Density  Density=1000  DensityUnits=kg/m^3  DoExposeReferenceFrame=on  SerializedFrames=<Frames/>  GraphicType=FromGeometry  MarkerShape=Sphere  MarkerSize=10  GraphicVisPropType=SimpleVisualProperties  GraphicDiffuseColor=smiData.Solid(3).color  GraphicSpecularColor=[0.5 0.5 0.5 1.0]  GraphicAmbientColor=[0.15 0.15 0.15 1.0]  GraphicEmissiveColor=[0.0 0.0 0.0 1.0]  GraphicShininess=75  GraphicOpacity=smiData.Solid(3).opacity
  F : PMIOPort  Side=Left
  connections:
  ReferenceFrame/RConn1 -- Solid/RConn1 -- F/RConn1

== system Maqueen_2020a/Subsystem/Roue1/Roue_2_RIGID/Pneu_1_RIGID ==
  ReferenceFrame : sm_lib/Frames and Transforms/Reference Frame
  Solid : sm_lib/Body Elements/File Solid  ExtGeomFileName=Pneu_Defaut_sldprt.STL  UnitType=Custom  ExtGeomFileUnits=mm  StepReaderType=HEX  ExportConvexHullGeometry=off  InertiaType=Custom  Mass=smiData.Solid(2).mass  MassUnits=kg  CenterOfMass=smiData.Solid(2).CoM  CenterOfMassUnits=mm  MomentsOfInertia=smiData.Solid(2).MoI  MomentsOfInertiaUnits=kg*mm^2  ProductsOfInertia=smiData.Solid(2).PoI  ProductsOfInertiaUnits=kg*mm^2  BasedOnType=Density  Density=1000  DensityUnits=kg/m^3  DoExposeReferenceFrame=on  SerializedFrames=<Frames/>  GraphicType=FromGeometry  MarkerShape=Sphere  MarkerSize=10  GraphicVisPropType=SimpleVisualProperties  GraphicDiffuseColor=smiData.Solid(2).color  GraphicSpecularColor=[0.5 0.5 0.5 1.0]  GraphicAmbientColor=[0.15 0.15 0.15 1.0]  GraphicEmissiveColor=[0.0 0.0 0.0 1.0]  GraphicShininess=75  GraphicOpacity=smiData.Solid(2).opacity
  F : PMIOPort  Side=Left
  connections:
  ReferenceFrame/RConn1 -- Solid/RConn1 -- F/RConn1

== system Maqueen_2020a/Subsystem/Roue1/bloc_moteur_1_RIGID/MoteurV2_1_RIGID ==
  ReferenceFrame : sm_lib/Frames and Transforms/Reference Frame
  Solid : sm_lib/Body Elements/File Solid  ExtGeomFileName=MoteurV2_Defaut_sldprt.STL  UnitType=Custom  ExtGeomFileUnits=mm  StepReaderType=HEX  ExportConvexHullGeometry=off  InertiaType=Custom  Mass=smiData.Solid(5).mass  MassUnits=kg  CenterOfMass=smiData.Solid(5).CoM  CenterOfMassUnits=mm  MomentsOfInertia=smiData.Solid(5).MoI  MomentsOfInertiaUnits=kg*mm^2  ProductsOfInertia=smiData.Solid(5).PoI  ProductsOfInertiaUnits=kg*mm^2  BasedOnType=Density  Density=1000  DensityUnits=kg/m^3  DoExposeReferenceFrame=on  SerializedFrames=<Frames/>  GraphicType=FromGeometry  MarkerShape=Sphere  MarkerSize=10  GraphicVisPropType=SimpleVisualProperties  GraphicDiffuseColor=smiData.Solid(5).color  GraphicSpecularColor=[0.5 0.5 0.5 1.0]  GraphicAmbientColor=[0.15 0.15 0.15 1.0]  GraphicEmissiveColor=[0.0 0.0 0.0 1.0]  GraphicShininess=75  GraphicOpacity=smiData.Solid(5).opacity
  F : PMIOPort  Side=Left
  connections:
  ReferenceFrame/RConn1 -- Solid/RConn1 -- F/RConn1

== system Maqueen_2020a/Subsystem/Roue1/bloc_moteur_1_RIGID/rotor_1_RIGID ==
  ReferenceFrame : sm_lib/Frames and Transforms/Reference Frame
  Solid : sm_lib/Body Elements/File Solid  ExtGeomFileName=rotor_Defaut_sldprt.STL  UnitType=Custom  ExtGeomFileUnits=m  StepReaderType=HEX  ExportConvexHullGeometry=off  InertiaType=Custom  Mass=smiData.Solid(6).mass  MassUnits=kg  CenterOfMass=smiData.Solid(6).CoM  CenterOfMassUnits=m  MomentsOfInertia=smiData.Solid(6).MoI  MomentsOfInertiaUnits=kg*m^2  ProductsOfInertia=smiData.Solid(6).PoI  ProductsOfInertiaUnits=kg*m^2  BasedOnType=Density  Density=1000  DensityUnits=kg/m^3  DoExposeReferenceFrame=on  SerializedFrames=<Frames/>  GraphicType=FromGeometry  MarkerShape=Sphere  MarkerSize=10  GraphicVisPropType=SimpleVisualProperties  GraphicDiffuseColor=smiData.Solid(6).color  GraphicSpecularColor=[0.5 0.5 0.5 1.0]  GraphicAmbientColor=[0.15 0.15 0.15 1.0]  GraphicEmissiveColor=[0.0 0.0 0.0 1.0]  GraphicShininess=75  GraphicOpacity=smiData.Solid(6).opacity
  F : PMIOPort  Side=Left
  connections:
  ReferenceFrame/RConn1 -- Solid/RConn1 -- F/RConn1

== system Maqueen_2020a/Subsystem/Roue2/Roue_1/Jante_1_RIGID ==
  ReferenceFrame : sm_lib/Frames and Transforms/Reference Frame
  Solid : sm_lib/Body Elements/File Solid  ExtGeomFileName=Jante_Defaut_sldprt.STL  UnitType=Custom  ExtGeomFileUnits=mm  StepReaderType=HEX  ExportConvexHullGeometry=off  InertiaType=Custom  Mass=smiData.Solid(3).mass  MassUnits=kg  CenterOfMass=smiData.Solid(3).CoM  CenterOfMassUnits=mm  MomentsOfInertia=smiData.Solid(3).MoI  MomentsOfInertiaUnits=kg*mm^2  ProductsOfInertia=smiData.Solid(3).PoI  ProductsOfInertiaUnits=kg*mm^2  BasedOnType=Density  Density=1000  DensityUnits=kg/m^3  DoExposeReferenceFrame=on  SerializedFrames=<Frames/>  GraphicType=FromGeometry  MarkerShape=Sphere  MarkerSize=10  GraphicVisPropType=SimpleVisualProperties  GraphicDiffuseColor=smiData.Solid(3).color  GraphicSpecularColor=[0.5 0.5 0.5 1.0]  GraphicAmbientColor=[0.15 0.15 0.15 1.0]  GraphicEmissiveColor=[0.0 0.0 0.0 1.0]  GraphicShininess=75  GraphicOpacity=smiData.Solid(3).opacity
  Transform : sm_lib/Frames and Transforms/Rigid Transform  TranslationMethod=Cartesian  TranslationStandardOffset=0  TranslationLengthUnit=mm  TranslationStandardAxis=+Z  TranslationCartesianOffset=smiData.RigidTransform(1).translation  TranslationROffset=0  TranslationROffsetUnits=m  TranslationZOffset=0  TranslationZOffsetUnits=m  TranslationThetaOffset=0  TranslationThetaOffsetUnits=deg  RotationMethod=ArbitraryAxis  RotationAngleUnits=rad  RotationStandardAxis=+Z  RotationAngle=smiData.RigidTransform(1).angle  RotationArbitraryAxis=smiData.RigidTransform(1).axis  FollAlignAxisA=+X  BaseAlignAxisA=+Y  FollAlignAxisB=+Y  BaseAlignAxisB=+Z  RotationSequenceAxes=FollowerAxes  RotationSequence=XYX  RotationSequenceAngles=[0 0 0]  RotationSequenceAnglesUnits=deg  RotationMatrix=[1 0 0; 0 1 0; 0 0 1]
  Transform1 : sm_lib/Frames and Transforms/Rigid Transform  TranslationMethod=Cartesian  TranslationStandardOffset=0  TranslationLengthUnit=mm  TranslationStandardAxis=+Z  TranslationCartesianOffset=smiData.RigidTransform(19).translation  TranslationROffset=0  TranslationROffsetUnits=m  TranslationZOffset=0  TranslationZOffsetUnits=m  TranslationThetaOffset=0  TranslationThetaOffsetUnits=deg  RotationMethod=ArbitraryAxis  RotationAngleUnits=rad  RotationStandardAxis=+Z  RotationAngle=smiData.RigidTransform(19).angle  RotationArbitraryAxis=smiData.RigidTransform(19).axis  FollAlignAxisA=+X  BaseAlignAxisA=+Y  FollAlignAxisB=+Y  BaseAlignAxisB=+Z  RotationSequenceAxes=FollowerAxes  RotationSequence=XYX  RotationSequenceAngles=[0 0 0]  RotationSequenceAnglesUnits=deg  RotationMatrix=[1 0 0; 0 1 0; 0 0 1]
  F2 : PMIOPort  Side=Left
  F1 : PMIOPort  Port=2  Side=Left
  F : PMIOPort  Port=3  Side=Left
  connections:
  ReferenceFrame/RConn1 -- Transform/LConn1 -- Transform1/LConn1 -- F2/RConn1 -- Solid/RConn1
  Transform/RConn1 -- F/RConn1
  Transform1/RConn1 -- F1/RConn1

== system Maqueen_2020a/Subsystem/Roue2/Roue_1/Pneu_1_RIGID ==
  ReferenceFrame : sm_lib/Frames and Transforms/Reference Frame
  Solid : sm_lib/Body Elements/File Solid  ExtGeomFileName=Pneu_Defaut_sldprt.STL  UnitType=Custom  ExtGeomFileUnits=mm  StepReaderType=HEX  ExportConvexHullGeometry=off  InertiaType=Custom  Mass=smiData.Solid(2).mass  MassUnits=kg  CenterOfMass=smiData.Solid(2).CoM  CenterOfMassUnits=mm  MomentsOfInertia=smiData.Solid(2).MoI  MomentsOfInertiaUnits=kg*mm^2  ProductsOfInertia=smiData.Solid(2).PoI  ProductsOfInertiaUnits=kg*mm^2  BasedOnType=Density  Density=1000  DensityUnits=kg/m^3  DoExposeReferenceFrame=on  SerializedFrames=<Frames/>  GraphicType=FromGeometry  MarkerShape=Sphere  MarkerSize=10  GraphicVisPropType=SimpleVisualProperties  GraphicDiffuseColor=smiData.Solid(2).color  GraphicSpecularColor=[0.5 0.5 0.5 1.0]  GraphicAmbientColor=[0.15 0.15 0.15 1.0]  GraphicEmissiveColor=[0.0 0.0 0.0 1.0]  GraphicShininess=75  GraphicOpacity=smiData.Solid(2).opacity
  Transform : sm_lib/Frames and Transforms/Rigid Transform  TranslationMethod=Cartesian  TranslationStandardOffset=0  TranslationLengthUnit=mm  TranslationStandardAxis=+Z  TranslationCartesianOffset=smiData.RigidTransform(2).translation  TranslationROffset=0  TranslationROffsetUnits=m  TranslationZOffset=0  TranslationZOffsetUnits=m  TranslationThetaOffset=0  TranslationThetaOffsetUnits=deg  RotationMethod=ArbitraryAxis  RotationAngleUnits=rad  RotationStandardAxis=+Z  RotationAngle=smiData.RigidTransform(2).angle  RotationArbitraryAxis=smiData.RigidTransform(2).axis  FollAlignAxisA=+X  BaseAlignAxisA=+Y  FollAlignAxisB=+Y  BaseAlignAxisB=+Z  RotationSequenceAxes=FollowerAxes  RotationSequence=XYX  RotationSequenceAngles=[0 0 0]  RotationSequenceAnglesUnits=deg  RotationMatrix=[1 0 0; 0 1 0; 0 0 1]
  F : PMIOPort  Side=Left
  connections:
  ReferenceFrame/RConn1 -- Solid/RConn1 -- Transform/LConn1
  Transform/RConn1 -- F/RConn1

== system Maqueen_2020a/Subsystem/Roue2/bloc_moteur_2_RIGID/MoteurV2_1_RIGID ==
  ReferenceFrame : sm_lib/Frames and Transforms/Reference Frame
  Solid : sm_lib/Body Elements/File Solid  ExtGeomFileName=MoteurV2_Defaut_sldprt.STL  UnitType=Custom  ExtGeomFileUnits=mm  StepReaderType=HEX  ExportConvexHullGeometry=off  InertiaType=Custom  Mass=smiData.Solid(5).mass  MassUnits=kg  CenterOfMass=smiData.Solid(5).CoM  CenterOfMassUnits=mm  MomentsOfInertia=smiData.Solid(5).MoI  MomentsOfInertiaUnits=kg*mm^2  ProductsOfInertia=smiData.Solid(5).PoI  ProductsOfInertiaUnits=kg*mm^2  BasedOnType=Density  Density=1000  DensityUnits=kg/m^3  DoExposeReferenceFrame=on  SerializedFrames=<Frames/>  GraphicType=FromGeometry  MarkerShape=Sphere  MarkerSize=10  GraphicVisPropType=SimpleVisualProperties  GraphicDiffuseColor=smiData.Solid(5).color  GraphicSpecularColor=[0.5 0.5 0.5 1.0]  GraphicAmbientColor=[0.15 0.15 0.15 1.0]  GraphicEmissiveColor=[0.0 0.0 0.0 1.0]  GraphicShininess=75  GraphicOpacity=smiData.Solid(5).opacity
  F : PMIOPort  Side=Left
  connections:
  ReferenceFrame/RConn1 -- Solid/RConn1 -- F/RConn1

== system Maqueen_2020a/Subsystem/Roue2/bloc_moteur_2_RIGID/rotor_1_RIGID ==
  ReferenceFrame : sm_lib/Frames and Transforms/Reference Frame
  Solid : sm_lib/Body Elements/File Solid  ExtGeomFileName=rotor_Defaut_sldprt.STL  UnitType=Custom  ExtGeomFileUnits=m  StepReaderType=HEX  ExportConvexHullGeometry=off  InertiaType=Custom  Mass=smiData.Solid(6).mass  MassUnits=kg  CenterOfMass=smiData.Solid(6).CoM  CenterOfMassUnits=m  MomentsOfInertia=smiData.Solid(6).MoI  MomentsOfInertiaUnits=kg*m^2  ProductsOfInertia=smiData.Solid(6).PoI  ProductsOfInertiaUnits=kg*m^2  BasedOnType=Density  Density=1000  DensityUnits=kg/m^3  DoExposeReferenceFrame=on  SerializedFrames=<Frames/>  GraphicType=FromGeometry  MarkerShape=Sphere  MarkerSize=10  GraphicVisPropType=SimpleVisualProperties  GraphicDiffuseColor=smiData.Solid(6).color  GraphicSpecularColor=[0.5 0.5 0.5 1.0]  GraphicAmbientColor=[0.15 0.15 0.15 1.0]  GraphicEmissiveColor=[0.0 0.0 0.0 1.0]  GraphicShininess=75  GraphicOpacity=smiData.Solid(6).opacity
  F : PMIOPort  Side=Left
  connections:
  ReferenceFrame/RConn1 -- Solid/RConn1 -- F/RConn1

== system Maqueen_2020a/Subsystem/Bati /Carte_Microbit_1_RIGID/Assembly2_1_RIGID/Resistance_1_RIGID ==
  ReferenceFrame : sm_lib/Frames and Transforms/Reference Frame
  Solid : sm_lib/Body Elements/File Solid  ExtGeomFileName=Resistance_Defaut_sldprt.STL  UnitType=Custom  ExtGeomFileUnits=mm  StepReaderType=HEX  ExportConvexHullGeometry=off  InertiaType=Custom  Mass=smiData.Solid(7).mass  MassUnits=kg  CenterOfMass=smiData.Solid(7).CoM  CenterOfMassUnits=mm  MomentsOfInertia=smiData.Solid(7).MoI  MomentsOfInertiaUnits=kg*mm^2  ProductsOfInertia=smiData.Solid(7).PoI  ProductsOfInertiaUnits=kg*mm^2  BasedOnType=Density  Density=1000  DensityUnits=kg/m^3  DoExposeReferenceFrame=on  SerializedFrames=<Frames/>  GraphicType=FromGeometry  MarkerShape=Sphere  MarkerSize=10  GraphicVisPropType=SimpleVisualProperties  GraphicDiffuseColor=smiData.Solid(7).color  GraphicSpecularColor=[0.5 0.5 0.5 1.0]  GraphicAmbientColor=[0.15 0.15 0.15 1.0]  GraphicEmissiveColor=[0.0 0.0 0.0 1.0]  GraphicShininess=75  GraphicOpacity=smiData.Solid(7).opacity
  F : PMIOPort  Side=Left
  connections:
  ReferenceFrame/RConn1 -- Solid/RConn1 -- F/RConn1

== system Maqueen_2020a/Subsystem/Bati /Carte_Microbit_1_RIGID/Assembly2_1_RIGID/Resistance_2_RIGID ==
  ReferenceFrame : sm_lib/Frames and Transforms/Reference Frame
  Solid : sm_lib/Body Elements/File Solid  ExtGeomFileName=Resistance_Defaut_sldprt.STL  UnitType=Custom  ExtGeomFileUnits=mm  StepReaderType=HEX  ExportConvexHullGeometry=off  InertiaType=Custom  Mass=smiData.Solid(7).mass  MassUnits=kg  CenterOfMass=smiData.Solid(7).CoM  CenterOfMassUnits=mm  MomentsOfInertia=smiData.Solid(7).MoI  MomentsOfInertiaUnits=kg*mm^2  ProductsOfInertia=smiData.Solid(7).PoI  ProductsOfInertiaUnits=kg*mm^2  BasedOnType=Density  Density=1000  DensityUnits=kg/m^3  DoExposeReferenceFrame=on  SerializedFrames=<Frames/>  GraphicType=FromGeometry  MarkerShape=Sphere  MarkerSize=10  GraphicVisPropType=SimpleVisualProperties  GraphicDiffuseColor=smiData.Solid(7).color  GraphicSpecularColor=[0.5 0.5 0.5 1.0]  GraphicAmbientColor=[0.15 0.15 0.15 1.0]  GraphicEmissiveColor=[0.0 0.0 0.0 1.0]  GraphicShininess=75  GraphicOpacity=smiData.Solid(7).opacity
  F : PMIOPort  Side=Left
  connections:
  ReferenceFrame/RConn1 -- Solid/RConn1 -- F/RConn1

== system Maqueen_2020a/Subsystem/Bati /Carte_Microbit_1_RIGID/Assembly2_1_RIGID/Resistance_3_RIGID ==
  ReferenceFrame : sm_lib/Frames and Transforms/Reference Frame
  Solid : sm_lib/Body Elements/File Solid  ExtGeomFileName=Resistance_Defaut_sldprt.STL  UnitType=Custom  ExtGeomFileUnits=mm  StepReaderType=HEX  ExportConvexHullGeometry=off  InertiaType=Custom  Mass=smiData.Solid(7).mass  MassUnits=kg  CenterOfMass=smiData.Solid(7).CoM  CenterOfMassUnits=mm  MomentsOfInertia=smiData.Solid(7).MoI  MomentsOfInertiaUnits=kg*mm^2  ProductsOfInertia=smiData.Solid(7).PoI  ProductsOfInertiaUnits=kg*mm^2  BasedOnType=Density  Density=1000  DensityUnits=kg/m^3  DoExposeReferenceFrame=on  SerializedFrames=<Frames/>  GraphicType=FromGeometry  MarkerShape=Sphere  MarkerSize=10  GraphicVisPropType=SimpleVisualProperties  GraphicDiffuseColor=smiData.Solid(7).color  GraphicSpecularColor=[0.5 0.5 0.5 1.0]  GraphicAmbientColor=[0.15 0.15 0.15 1.0]  GraphicEmissiveColor=[0.0 0.0 0.0 1.0]  GraphicShininess=75  GraphicOpacity=smiData.Solid(7).opacity
  F : PMIOPort  Side=Left
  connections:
  ReferenceFrame/RConn1 -- Solid/RConn1 -- F/RConn1

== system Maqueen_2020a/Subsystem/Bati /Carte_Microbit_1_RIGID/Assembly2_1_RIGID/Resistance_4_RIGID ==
  ReferenceFrame : sm_lib/Frames and Transforms/Reference Frame
  Solid : sm_lib/Body Elements/File Solid  ExtGeomFileName=Resistance_Defaut_sldprt.STL  UnitType=Custom  ExtGeomFileUnits=mm  StepReaderType=HEX  ExportConvexHullGeometry=off  InertiaType=Custom  Mass=smiData.Solid(7).mass  MassUnits=kg  CenterOfMass=smiData.Solid(7).CoM  CenterOfMassUnits=mm  MomentsOfInertia=smiData.Solid(7).MoI  MomentsOfInertiaUnits=kg*mm^2  ProductsOfInertia=smiData.Solid(7).PoI  ProductsOfInertiaUnits=kg*mm^2  BasedOnType=Density  Density=1000  DensityUnits=kg/m^3  DoExposeReferenceFrame=on  SerializedFrames=<Frames/>  GraphicType=FromGeometry  MarkerShape=Sphere  MarkerSize=10  GraphicVisPropType=SimpleVisualProperties  GraphicDiffuseColor=smiData.Solid(7).color  GraphicSpecularColor=[0.5 0.5 0.5 1.0]  GraphicAmbientColor=[0.15 0.15 0.15 1.0]  GraphicEmissiveColor=[0.0 0.0 0.0 1.0]  GraphicShininess=75  GraphicOpacity=smiData.Solid(7).opacity
  F : PMIOPort  Side=Left
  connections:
  ReferenceFrame/RConn1 -- Solid/RConn1 -- F/RConn1

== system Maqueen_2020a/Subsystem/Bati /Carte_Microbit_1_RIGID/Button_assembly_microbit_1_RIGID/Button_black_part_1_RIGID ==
  ReferenceFrame : sm_lib/Frames and Transforms/Reference Frame
  Solid : sm_lib/Body Elements/File Solid  ExtGeomFileName=Button black part_Defaut_sldprt.STL  UnitType=Custom  ExtGeomFileUnits=mm  StepReaderType=HEX  ExportConvexHullGeometry=off  InertiaType=Custom  Mass=smiData.Solid(23).mass  MassUnits=kg  CenterOfMass=smiData.Solid(23).CoM  CenterOfMassUnits=mm  MomentsOfInertia=smiData.Solid(23).MoI  MomentsOfInertiaUnits=kg*mm^2  ProductsOfInertia=smiData.Solid(23).PoI  ProductsOfInertiaUnits=kg*mm^2  BasedOnType=Density  Density=1000  DensityUnits=kg/m^3  DoExposeReferenceFrame=on  SerializedFrames=<Frames/>  GraphicType=FromGeometry  MarkerShape=Sphere  MarkerSize=10  GraphicVisPropType=SimpleVisualProperties  GraphicDiffuseColor=smiData.Solid(23).color  GraphicSpecularColor=[0.5 0.5 0.5 1.0]  GraphicAmbientColor=[0.15 0.15 0.15 1.0]  GraphicEmissiveColor=[0.0 0.0 0.0 1.0]  GraphicShininess=75  GraphicOpacity=smiData.Solid(23).opacity
  F : PMIOPort  Side=Left
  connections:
  ReferenceFrame/RConn1 -- Solid/RConn1 -- F/RConn1

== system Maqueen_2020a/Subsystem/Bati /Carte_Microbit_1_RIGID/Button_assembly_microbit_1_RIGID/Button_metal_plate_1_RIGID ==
  ReferenceFrame : sm_lib/Frames and Transforms/Reference Frame
  Solid : sm_lib/Body Elements/File Solid  ExtGeomFileName=Button metal plate_Defaut_sldprt.STL  UnitType=Custom  ExtGeomFileUnits=mm  StepReaderType=HEX  ExportConvexHullGeometry=off  InertiaType=Custom  Mass=smiData.Solid(25).mass  MassUnits=kg  CenterOfMass=smiData.Solid(25).CoM  CenterOfMassUnits=mm  MomentsOfInertia=smiData.Solid(25).MoI  MomentsOfInertiaUnits=kg*mm^2  ProductsOfInertia=smiData.Solid(25).PoI  ProductsOfInertiaUnits=kg*mm^2  BasedOnType=Density  Density=1000  DensityUnits=kg/m^3  DoExposeReferenceFrame=on  SerializedFrames=<Frames/>  GraphicType=FromGeometry  MarkerShape=Sphere  MarkerSize=10  GraphicVisPropType=SimpleVisualProperties  GraphicDiffuseColor=smiData.Solid(25).color  GraphicSpecularColor=[0.5 0.5 0.5 1.0]  GraphicAmbientColor=[0.15 0.15 0.15 1.0]  GraphicEmissiveColor=[0.0 0.0 0.0 1.0]  GraphicShininess=75  GraphicOpacity=smiData.Solid(25).opacity
  F : PMIOPort  Side=Left
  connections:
  ReferenceFrame/RConn1 -- Solid/RConn1 -- F/RConn1

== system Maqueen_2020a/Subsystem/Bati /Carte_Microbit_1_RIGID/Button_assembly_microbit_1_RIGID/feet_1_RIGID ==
  ReferenceFrame : sm_lib/Frames and Transforms/Reference Frame
  Solid : sm_lib/Body Elements/File Solid  ExtGeomFileName=feet_Defaut_sldprt.STL  UnitType=Custom  ExtGeomFileUnits=mm  StepReaderType=HEX  ExportConvexHullGeometry=off  InertiaType=Custom  Mass=smiData.Solid(24).mass  MassUnits=kg  CenterOfMass=smiData.Solid(24).CoM  CenterOfMassUnits=mm  MomentsOfInertia=smiData.Solid(24).MoI  MomentsOfInertiaUnits=kg*mm^2  ProductsOfInertia=smiData.Solid(24).PoI  ProductsOfInertiaUnits=kg*mm^2  BasedOnType=Density  Density=1000  DensityUnits=kg/m^3  DoExposeReferenceFrame=on  SerializedFrames=<Frames/>  GraphicType=FromGeometry  MarkerShape=Sphere  MarkerSize=10  GraphicVisPropType=SimpleVisualProperties  GraphicDiffuseColor=smiData.Solid(24).color  GraphicSpecularColor=[0.5 0.5 0.5 1.0]  GraphicAmbientColor=[0.15 0.15 0.15 1.0]  GraphicEmissiveColor=[0.0 0.0 0.0 1.0]  GraphicShininess=75  GraphicOpacity=smiData.Solid(24).opacity
  F : PMIOPort  Side=Left
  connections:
  ReferenceFrame/RConn1 -- Solid/RConn1 -- F/RConn1

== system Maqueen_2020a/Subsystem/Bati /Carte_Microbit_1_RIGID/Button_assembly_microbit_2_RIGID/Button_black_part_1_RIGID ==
  ReferenceFrame : sm_lib/Frames and Transforms/Reference Frame
  Solid : sm_lib/Body Elements/File Solid  ExtGeomFileName=Button black part_Defaut_sldprt.STL  UnitType=Custom  ExtGeomFileUnits=mm  StepReaderType=HEX  ExportConvexHullGeometry=off  InertiaType=Custom  Mass=smiData.Solid(23).mass  MassUnits=kg  CenterOfMass=smiData.Solid(23).CoM  CenterOfMassUnits=mm  MomentsOfInertia=smiData.Solid(23).MoI  MomentsOfInertiaUnits=kg*mm^2  ProductsOfInertia=smiData.Solid(23).PoI  ProductsOfInertiaUnits=kg*mm^2  BasedOnType=Density  Density=1000  DensityUnits=kg/m^3  DoExposeReferenceFrame=on  SerializedFrames=<Frames/>  GraphicType=FromGeometry  MarkerShape=Sphere  MarkerSize=10  GraphicVisPropType=SimpleVisualProperties  GraphicDiffuseColor=smiData.Solid(23).color  GraphicSpecularColor=[0.5 0.5 0.5 1.0]  GraphicAmbientColor=[0.15 0.15 0.15 1.0]  GraphicEmissiveColor=[0.0 0.0 0.0 1.0]  GraphicShininess=75  GraphicOpacity=smiData.Solid(23).opacity
  F : PMIOPort  Side=Left
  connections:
  ReferenceFrame/RConn1 -- Solid/RConn1 -- F/RConn1
